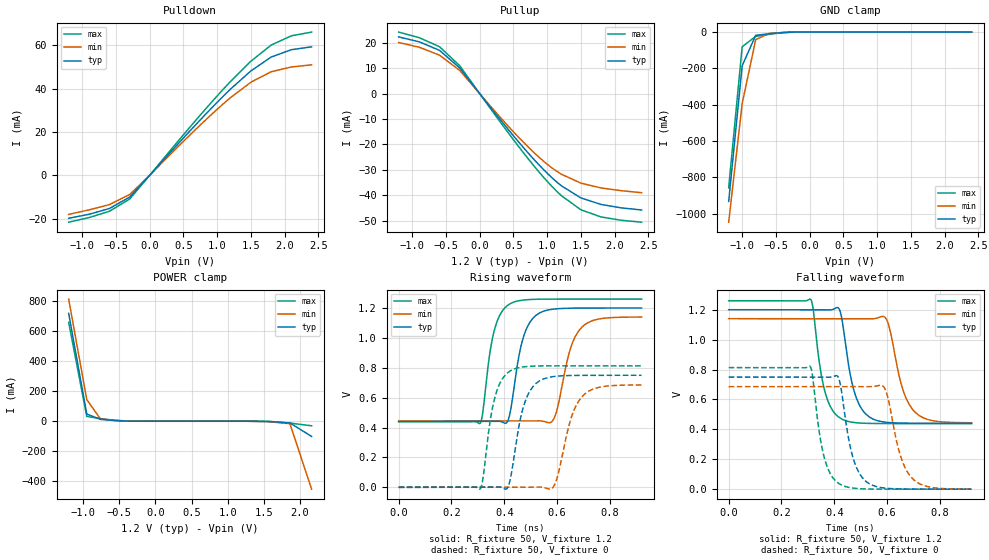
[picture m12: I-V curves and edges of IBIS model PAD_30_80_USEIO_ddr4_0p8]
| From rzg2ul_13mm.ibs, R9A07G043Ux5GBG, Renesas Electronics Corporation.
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[Model] PAD_30_80_USEIO_ddr4_0p8
Model_type I/O
Polarity   Non-Inverting
Vinl = 0.8670
Vinh = 1.0530
Vmeas= 0.960
| Capacitance   typ   min   max
C_comp   2.102e-12   2.013e-12   2.216e-12
[Model Spec]
| Subparameter   typ   min   max
Vmeas   0.960   0.912   1.008
Vinh   1.0530   1.0050   1.1010
Vinl   0.8670   0.8190   0.9150
| Variables   typ   min   max
[GND Clamp Reference]   0   0   0
[POWER Clamp Reference]   1.2   1.14   1.26
[Pulldown Reference]   0   0   0
[Pullup Reference]   1.2   1.14   1.26
[Temperature Range]   25   125   -40
[Voltage Range]   1.2   1.14   1.26
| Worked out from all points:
|   slope of the pulldown table from 0 to 0.18 V, typ, clamps not added: 28.9 ohm
|   slope of the pullup table from 0 to 0.18 V, typ, clamps not added: 29.6 ohm
|   GND clamp passes 1 mA (typ) near -0.30 V on its own axis
|   POWER clamp passes 1 mA (typ) near -0.38 V on its own axis
|   rising waveform, R_fixture 50, V_fixture 1.2: 20-80 % time 50.2ps typ, 58.4ps min, 44.3ps max; typ from 0.44 V to 1.2 V
|   rising waveform, R_fixture 50, V_fixture 0: 20-80 % time 52.3ps typ, 61.8ps min, 46.1ps max; typ from 0 V to 0.75 V
|   falling waveform, R_fixture 50, V_fixture 1.2: 20-80 % time 51ps typ, 60.1ps min, 46.1ps max; typ from 1.2 V to 0.44 V
|   falling waveform, R_fixture 50, V_fixture 0: 20-80 % time 50.7ps typ, 59.1ps min, 45.9ps max; typ from 0.749 V to 0 V
[GND Clamp]
| Voltage   I(typ)   I(min)   I(max)
-1.2V     -932.7mA   -1.047A    -857.4mA
-1V       -185.5mA   -394.3mA   -80.64mA
-800mV    -17.89mA   -41.9mA    -23.65mA
-600mV    -9.04mA    -7.411mA   -12.44mA
-400mV    -2.454mA   -2.378mA   -3.185mA
2.4V      0A         0A         0A
[POWER Clamp]
| Voltage   I(typ)   I(min)   I(max)
-1.2V     719.7mA    815.2mA    660.1mA
-950mV    48.1mA     144.6mA    32.07mA
-760mV    12.41mA    14.91mA    17.11mA
-360mV    527.4uA    791.2uA    575.5uA
1.26V     -115.5nA   -12.89uA   -796.6pA
1.56V     -1.53mA    -2.776mA   -549.4uA
1.86V     -11.39mA   -16.33mA   -12.44mA
2.16V     -101.5mA   -453.2mA   -30.39mA
[Pulldown]
| Voltage   I(typ)   I(min)   I(max)
-1.2V     -19.8mA    -18mA      -21.6mA
-895mV    -17.93mA   -15.9mA    -19.45mA
-595mV    -15.26mA   -13.48mA   -16.54mA
-295mV    -9.988mA   -8.815mA   -10.9mA
500mV     17.21mA    15.66mA    18.69mA
905mV     30.65mA    27.77mA    33.32mA
1.21V     40.14mA    36.16mA    43.71mA
1.5V      48.18mA    42.97mA    52.66mA
1.8V      54.57mA    47.8mA     60.1mA
2.1V      57.97mA    50mA       64.38mA
2.4V      59.3mA     51mA       66.1mA
[Pullup]
| Voltage   I(typ)   I(min)   I(max)
-1.2V     22.3mA     20.1mA     24.2mA
-895mV    20.36mA    18.24mA    22mA
-595mV    17.02mA    15.13mA    18.44mA
-295mV    10.08mA    9.108mA    10.95mA
300mV     -10.08mA   -9.168mA   -10.99mA
650mV     -21.28mA   -19.18mA   -23.31mA
955mV     -30.11mA   -26.78mA   -33.15mA
1.21V     -36.25mA   -31.71mA   -40.14mA
1.5V      -41.05mA   -35.23mA   -45.72mA
1.8V      -43.63mA   -37.14mA   -48.55mA
2.1V      -44.97mA   -38.2mA    -49.85mA
2.4V      -45.8mA    -39mA      -50.6mA
[Ramp]
dV/dt_r   0.4557/5.017e-11   0.4176/5.841e-11   0.4928/4.434e-11
dV/dt_f   0.4497/5.073e-11   0.4111/5.907e-11   0.4878/4.590e-11
R_load= 50
[Rising Waveform]
R_fixture = 50
V_fixture = 1.2
V_fixture_min = 1.14
V_fixture_max = 1.26
| Time   V(typ)   V(min)   V(max)
0s        440.5mV    443.8mV    438.7mV
309ps     440.5mV    443.8mV    429.6mV
358ps     440.9mV    443.8mV    1.021V
408ps     430.3mV    443.8mV    1.211V
479ps     1.04V      443.7mV    1.255V
575ps     1.19V      433.3mV    1.26V
600ps     1.195V     520.7mV    1.26V
650ps     1.199V     925.4mV    1.26V
684ps     1.2V       1.052V     1.26V
920ps     1.2V       1.14V      1.26V
[Rising Waveform]
R_fixture = 50
V_fixture = 0
V_fixture_min = 0
V_fixture_max = 0
| Time   V(typ)   V(min)   V(max)
0s        80.42nV    3.391uV    13.78nV
309ps     619.3nV    3.136uV    -10.31mV
357ps     375.7uV    2.79uV     547.5mV
409ps     -10.07mV   19.9uV     761.8mV
486ps     606.3mV    -1.655uV   808.7mV
576ps     738.5mV    -10.95mV   813mV
600ps     744.2mV    62.21mV    813.2mV
656ps     748.6mV    479.2mV    813.3mV
692ps     749.4mV    601.6mV    813.3mV
920ps     749.7mV    685.3mV    813.3mV
[Falling Waveform]
R_fixture = 50
V_fixture = 1.2
V_fixture_min = 1.14
V_fixture_max = 1.26
| Time   V(typ)   V(min)   V(max)
0s        1.2V       1.14V      1.26V
311ps     1.2V       1.14V      1.268V
359ps     1.2V       1.14V      691.3mV
415ps     1.212V     1.14V      484.1mV
463ps     742.9mV    1.14V      448.9mV
489ps     585.6mV    1.14V      443.1mV
589ps     448.9mV    1.153V     438.6mV
658ps     441.4mV    675.4mV    438.4mV
700ps     440.5mV    525.9mV    438.4mV
920ps     440.2mV    444.1mV    438.4mV
[Falling Waveform]
R_fixture = 50
V_fixture = 0
V_fixture_min = 0
V_fixture_max = 0
| Time   V(typ)   V(min)   V(max)
0s        749.5mV    685.4mV    812.9mV
309ps     749.5mV    685.4mV    819mV
358ps     749.2mV    685.4mV    238.8mV
411ps     757.2mV    685.4mV    46.37mV
482ps     153mV      685.4mV    5.016mV
579ps     9.892mV    694.2mV    204.2uV
600ps     5.303mV    632mV      100.5uV
654ps     1.176mV    204.4mV    20.98uV
694ps     338.4uV    74.44mV    3.761uV
920ps     319.5nV    250.1uV    15.29nV
[Add Submodel]
| Submodel Name Mode
PAD_30_80_0p8_T Non-Driving
